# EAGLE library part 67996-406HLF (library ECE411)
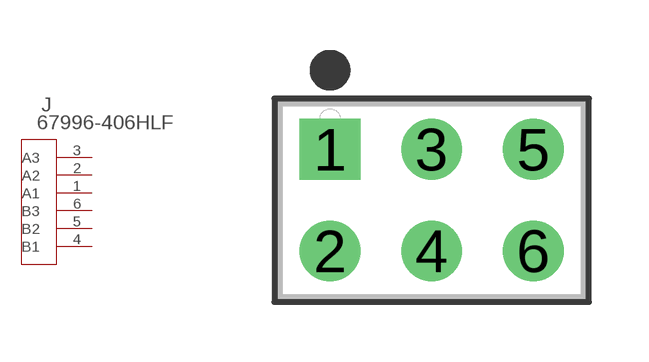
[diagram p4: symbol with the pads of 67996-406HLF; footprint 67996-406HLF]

Designator prefix J

## 67996-406HLF (MANUFACTURER_PART_NUMBER: 67996406HLF; VENDOR: Amphenol FCI)  [67996-406HLF]
1  A1  pas
2  A2  pas
3  A3  pas
4  B1  pas
5  B2  pas
6  B3  pas

## Footprint 67996-406HLF (pad centres in mm)
drill 0.965 pad 1.524 square: 1 -5.08,2.54
drill 1.016 pad 1.524: 2 -5.08,0; 3 -2.54,2.54; 4 -2.54,0; 5 0,2.54; 6 0,0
